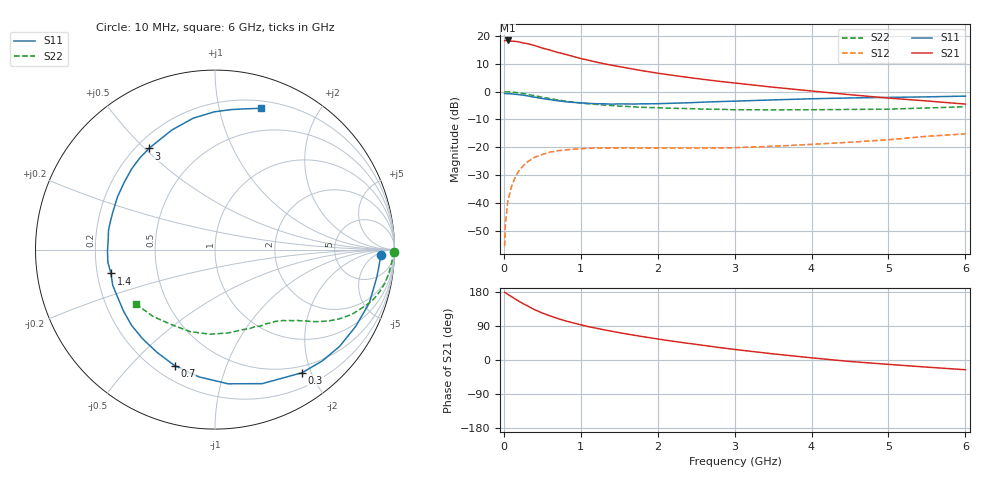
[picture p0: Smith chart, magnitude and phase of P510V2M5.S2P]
! SIEMENS Small Signal Semiconductors
! BFP183
! Si NPN RF Bipolar Junction Transistor in SOT143
! VCE = 10 V  IC = 2.5 mA
! Common Emitter S-Parameters:  March  1996
# GHz  S  MA  R  50
!  f  S11  S21  S12  S22
! GHz  MAG  ANG  MAG  ANG  MAG  ANG  MAG  ANG
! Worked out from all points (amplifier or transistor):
!   36 points, 10 MHz to 6 GHz, reference 50 ohm
!   highest |S21| = 18.3 dB at 50 MHz (marker M1)
!   |S21| within 3 dB of that: start of sweep to 538 MHz
!   unconditionally stable (mu >= 1): 2.058 GHz to 5.84 GHz
!   at 250 MHz: K = 0.13, MSG = 22.0 dB, |S12| = -26.7 dB
!   at 1.4 GHz: K = 0.71, MSG = 14.8 dB, |S12| = -20.2 dB
!   at 6 GHz: K = 0.96, MSG = 5.3 dB, |S12| = -15.2 dB
!   S11 on the Smith chart (normalised r, x): 10 MHz: 22, -10; 300 MHz: 0.40, -1.87; 700 MHz: 0.28, -0.67; 1.4 GHz: 0.26, -0.11; 3 GHz: 0.25, +0.52; 6 GHz: 0.27, +1.34
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0.01  0.9267 -1.9  8.14 178.7  0.0017 84.1  0.9958 -0.7
0.02  0.9208 -3.9  8.188 177.8  0.0041 84.6  0.9891 -1.5
0.05  0.9149 -9.5  8.224 173.4  0.0105 85.0  0.9887 -3.7
0.15  0.8933 -28.5  7.923 160.7  0.0298 73.6  0.9654 -11.1
0.2  0.8793 -37.7  7.738 154.5  0.0388 68.9  0.9462 -14.5
0.25  0.8614 -46.1  7.421 148.7  0.0465 64.4  0.9239 -17.6
0.3  0.8403 -54.7  7.238 143.6  0.0542 59.8  0.8965 -20.3
0.4  0.7918 -70.6  6.676 132.8  0.0664 52.1  0.8441 -25.3
0.5  0.7513 -84.4  6.012 124.0  0.0748 45.2  0.7919 -29.2
0.6  0.715 -97.1  5.525 116.5  0.0822 40.2  0.7479 -32.1
0.7  0.6845 -109.2  5.026 109.6  0.0869 35.5  0.7078 -34.5
0.8  0.6576 -119.4  4.642 103.3  0.0901 31.8  0.674 -36.5
0.9  0.6398 -129.2  4.265 98.0  0.0928 28.9  0.6441 -38.1
1.1  0.6143 -146.0  3.64 88.0  0.0961 23.9  0.6022 -40.9
1.4  0.5949 -167.1  2.964 76.0  0.0979 18.8  0.5617 -44.9
1.7  0.5975 174.8  2.497 65.2  0.0972 16.7  0.5298 -48.8
2.2  0.6179 151.5  1.948 49.4  0.097 15.5  0.5004 -55.9
3  0.6731 123.1  1.423 27.9  0.0988 18.2  0.4727 -70.3
3.5  0.7085 109.8  1.196 16.2  0.1046 20.7  0.4702 -80.8
4.5  0.7676 90.3  0.878 -3.9  0.1236 23.5  0.4777 -106.9
5.5  0.8032 77.6  0.678 -18.8  0.1579 23.3  0.5077 -132.8
6  0.828 71.9  0.596 -25.7  0.1746 20.2  0.534 -145.2
